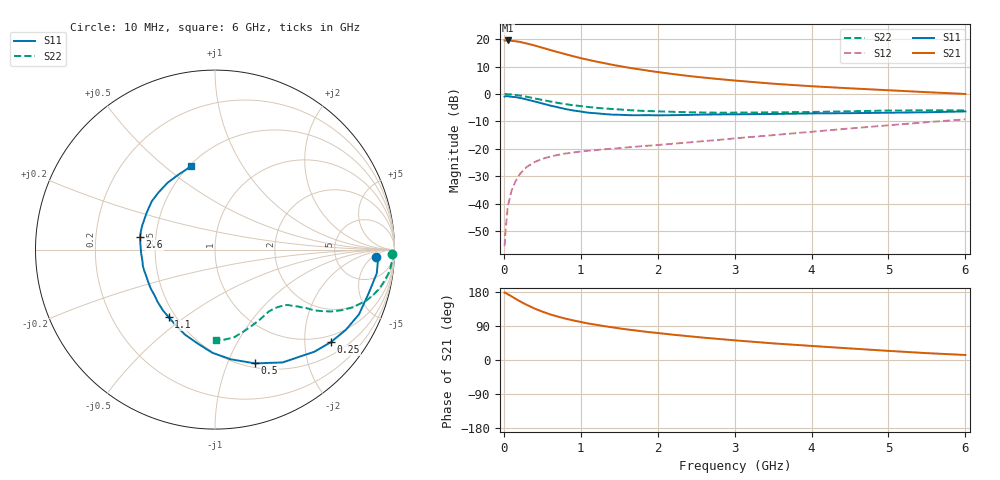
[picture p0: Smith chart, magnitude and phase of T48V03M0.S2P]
! Infineon Technologies  Discrete & RF Semiconductors
! BFR182T
! Si NPN RF Bipolar Junction Transistor in SC75
! VCE = 8 V  IC = 3 mA
! Common Emitter S-Parameters:  October  1999
# GHz  S  MA  R  50
!  f  S11  S21  S12  S22
! GHz  MAG  ANG  MAG  ANG  MAG  ANG  MAG  ANG
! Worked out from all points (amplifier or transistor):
!   36 points, 10 MHz to 6 GHz, reference 50 ohm
!   highest |S21| = 19.5 dB at 50 MHz (marker M1)
!   |S21| within 3 dB of that: start of sweep to 544.5 MHz
!   unconditionally stable (mu >= 1): 1.82 GHz to 4.299 GHz
!   at 250 MHz: K = 0.19, MSG = 23.3 dB, |S12| = -27.9 dB
!   at 1.4 GHz: K = 0.87, MSG = 15.3 dB, |S12| = -19.9 dB
!   at 6 GHz: K = 0.84, MSG = 4.6 dB, |S12| = -9.2 dB
!   lowest NFmin = 1.10 dB at 450 MHz
!   S11 on the Smith chart (normalised r, x): 10 MHz: 16, -7; 250 MHz: 0.81, -2.64; 500 MHz: 0.55, -1.26; 1.1 GHz: 0.46, -0.44; 2.6 GHz: 0.41, +0.07; 6 GHz: 0.51, +0.62
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0.01  0.9002 -2.7  9.434 177.8  0.0017 88.6  0.986 -1.5
0.02  0.911 -1.9  9.426 177.6  0.0029 90.2  0.996 -1.4
0.05  0.911 -8.3  9.438 173.7  0.0087 86.2  0.9888 -3.6
0.15  0.8796 -24.2  9.145 161.8  0.0256 77.2  0.9614 -10.3
0.2  0.8552 -31.5  8.93 156.0  0.0337 74.7  0.9418 -13.3
0.25  0.8262 -38.6  8.611 150.5  0.0405 69.5  0.9157 -16.1
0.3  0.7939 -45.8  8.3 145.3  0.0473 66.7  0.89 -18.6
0.4  0.7327 -59.1  7.642 135.7  0.0578 60.9  0.832 -22.8
0.5  0.6721 -70.6  6.964 127.7  0.0661 56.5  0.7798 -25.7
0.6  0.6176 -81.8  6.346 120.5  0.0724 53.1  0.7324 -28.1
0.7  0.5755 -91.4  5.794 114.6  0.0778 50.8  0.69 -29.8
0.8  0.5327 -100.3  5.32 109.2  0.0826 49.1  0.6551 -31.2
0.9  0.503 -109.2  4.878 104.5  0.086 48.0  0.6245 -32.1
1.1  0.4568 -124.3  4.187 96.2  0.093 46.8  0.5802 -33.7
1.3  0.4327 -137.5  3.662 89.5  0.0987 46.7  0.5469 -35.2
1.6  0.4133 -154.4  3.051 80.7  0.1066 48.0  0.5119 -37.1
2.2  0.4122 -177.6  2.308 66.8  0.1247 51.6  0.4745 -42.4
2.6  0.4232 170.7  1.989 58.9  0.1389 54.0  0.461 -46.8
3.5  0.4329 151.4  1.541 43.9  0.1784 57.4  0.4632 -57.6
4.5  0.4479 134.4  1.27 30.5  0.2361 58.0  0.4843 -71.1
5.5  0.4655 115.4  1.08 18.1  0.307 55.2  0.5044 -83.8
6  0.4824 106.0  1.002 13.2  0.3464 52.4  0.5026 -89.3
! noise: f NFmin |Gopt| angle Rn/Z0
0.45  1.1  0.37  30  0.33
0.9  1.2  0.35  61  0.26
1.8  1.85  0.27  133  0.2
